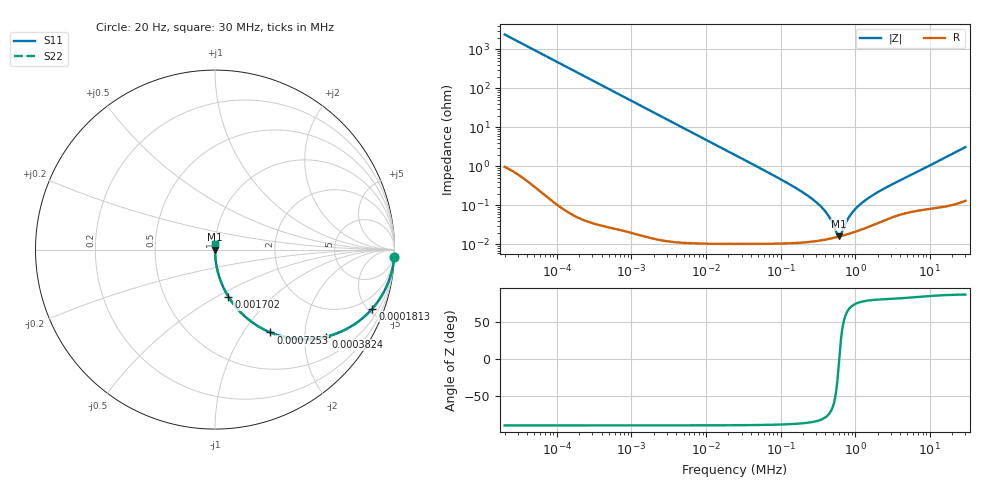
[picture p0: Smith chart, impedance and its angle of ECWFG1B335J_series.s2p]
!  *** S-Parameter ***
!  Copyright (C) Panasonic Industry
!  Plastic Film Capacitor (ECWFG)
!  Parts No. ECWFG1B335J
!  Connection Mode : Series
!  1  o---||---o  2
!  GND o--------o GND
!  Conditions : Temperature = 20   DC Bias = 0 V
! Frequency Range : 20 Hz  -  30 MHz  [ 401 Steps ]
# Hz S RI R 50
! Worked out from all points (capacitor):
!   401 points, 20 Hz to 30 MHz, reference 50 ohm
!   read as one part in series: C = 3.29 uF near 21.47 Hz
!   lowest |Z| = 16.1 mohm at 600.8 kHz (marker M1)
!   series resonance near 611.1 kHz, so ESL is about 21 nH
!   S11 on the Smith chart (normalised r, x): 20 Hz: 1, -48; 181.3 Hz: 1.00, -5.34; 382.4 Hz: 1.00, -2.53; 725.3 Hz: 1.00, -1.34; 1.702 kHz: 1.00, -0.57; 30 MHz: 1.00, +0.06
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20  0.9983 -0.0412  0.00172 0.0412  0.00172 0.0412  0.9983 -0.0412
66.98811  0.9812 -0.1357  0.0188 0.1357  0.0188 0.1357  0.9812 -0.1357
181.2693  0.8771 -0.3282  0.1229 0.3282  0.1229 0.3282  0.8771 -0.3282
216.5336  0.8334 -0.3725  0.1666 0.3725  0.1666 0.3725  0.8334 -0.3725
382.445  0.616 -0.4862  0.384 0.4862  0.384 0.4862  0.616 -0.4862
725.2589  0.3086 -0.4617  0.6914 0.4617  0.6914 0.4617  0.3086 -0.4617
1111.158  0.1598 -0.3662  0.8402 0.3662  0.8402 0.3662  0.1598 -0.3662
1702.388  0.075 -0.2632  0.925 0.2632  0.925 0.2632  0.075 -0.2632
2344.34  0.0411 -0.1982  0.9589 0.1982  0.9589 0.1982  0.0411 -0.1982
6343.763  0.0059 -0.0759  0.9941 0.0759  0.9941 0.0759  0.0059 -0.0759
24494.9  0.000493 -0.0197  0.9995 0.0197  0.9995 0.0197  0.000493 -0.0197
125697.3  0.00012 -0.00368  0.9999 0.00368  0.9999 0.00368  0.00012 -0.00368
265198.4  0.000121 -0.00147  0.9999 0.00147  0.9999 0.00147  0.000121 -0.00147
406306.4  0.000135 -0.000655  0.9999 0.000655  0.9999 0.000655  0.000135 -0.000655
559520.1  0.000154 -0.000136  0.9998 0.000136  0.9998 0.000136  0.000154 -0.000136
600753.3  0.000159 -2.6e-05  0.9998 2.6e-05  0.9998 2.6e-05  0.000159 -2.6e-05
645025.1  0.000165 8.36e-05  0.9998 -8.36e-05  0.9998 -8.36e-05  0.000165 8.36e-05
857232.1  0.000193 0.000526  0.9998 -0.000526  0.9998 -0.000526  0.000193 0.000526
1061060  0.000221 0.000877  0.9998 -0.000877  0.9998 -0.000877  0.000221 0.000877
1568853  0.000293 0.00161  0.9997 -0.00161  0.9997 -0.00161  0.000293 0.00161
2871218  0.000476 0.00317  0.9995 -0.00317  0.9995 -0.00317  0.000476 0.00317
3e7  0.0023 0.0313  0.9977 -0.0313  0.9977 -0.0313  0.0023 0.0313
